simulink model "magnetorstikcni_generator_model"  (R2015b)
settings: Solver=VariableStepAuto  StartTime=0.0  StopTime=1  FixedStep=1e-3  RelTol=1e-3
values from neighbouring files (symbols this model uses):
  A = (pi*d_terf^2)/4    (= 5.02654824574e-05)    [parametry_magneto.m]    (also in P_016_80_parametry.m = 0.00020106192983)
  A_c = ((pi*D_c^2)/4)-((pi*d_c^2)/4)    [parametry_magneto.m]
  b = 2*b_p*m_t*ome    [parametry_magneto.m]    (also in P_016_80_parametry.m = 415.611533333)
  b_amp = 2*0.02*m_amp*ome_amp    (= 29.2857142857)    [parametry_magneto.m]    (also in piezoelektricky_genarator_parametry.m = 3.90920092413)
  d33 = 2e-9    (= 2e-09)    [parametry_magneto.m]    (also in P_016_80_parametry.m = 6.5e-10)
  delta_x = 4e-4    (= 0.0004)    [parametry_magneto.m]    (also in piezoelektricky_genarator_parametry.m)
  k = E*A/l_terf    (= 1005309649.15)    [parametry_magneto.m]    (also in P_016_80_parametry.m = 56000000)
  k_amp = F_in/delta_x    (= 6821500)    [parametry_magneto.m]    (also in piezoelektricky_genarator_parametry.m)
  L = (perm*(N_c^2)*A_c)/l_c    [parametry_magneto.m]
  l_terf = 0.025    [parametry_magneto.m]
  m = m_t+m_amp    (= 2.02300536849)    [parametry_magneto.m]    (also in piezoelektricky_genarator_parametry.m = m_eff+m_amp; P_016_80_parametry.m = 0.1804)
  N_c = N_c_row*floor(N_c/N_c_row)    [parametry_magneto.m]
  perm = 6.29e-6    (= 6.29e-06)    [parametry_magneto.m]
  Rc = 4*(ro_Cu*l_d)/(pi*d_d^2)    [parametry_magneto.m]
  Rz = 250    [parametry_magneto.m]

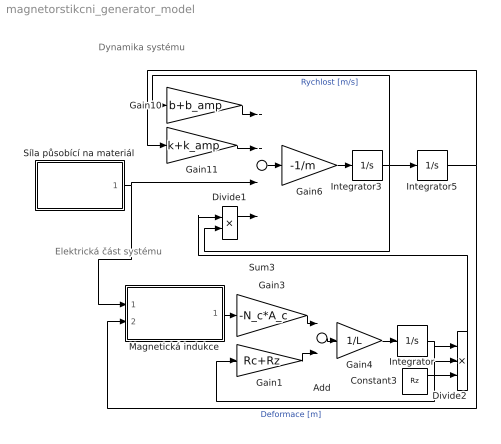
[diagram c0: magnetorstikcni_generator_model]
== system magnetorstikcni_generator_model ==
  note: Dynamika systému
  note: Elektrická část systému
  Add : Sum  Inputs=+-
  Constant3 : Constant  Value=Rz
  Divide1 : Product  Inputs=*/
  Divide2 : Product  Inputs=***
  Gain1 : Gain  Gain=Rc+Rz
  Gain10 : Gain  Gain=b+b_amp
  Gain11 : Gain  Gain=k+k_amp
  Gain3 : Gain  Gain=-N_c*A_c
  Gain4 : Gain  Gain=1/L
  Gain6 : Gain  Gain=-1/m
  Integrator : Integrator
  Integrator3 : Integrator  InitialCondition=1.5e-5
  Integrator5 : Integrator
  Magnetická indukce : Subsystem
  Sum3 : Sum  Inputs=++--
  Síla působící na materiál : Subsystem
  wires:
  Gain6/1 -> Integrator3/1
  Sum3/1 -> Gain6/1
  Gain10/1 -> Sum3/1
  Integrator3/1 -> Integrator5/1, Gain10/1, Divide1/2  "Rychlost [m/s]"
  Gain11/1 -> Sum3/2
  Integrator5/1 -> Gain11/1, Magnetická indukce/2(Deformace)  "Deformace [m]"
  Gain3/1 -> Add/1
  Add/1 -> Gain4/1
  Gain1/1 -> Add/2
  Gain4/1 -> Integrator/1
  Integrator/1 -> Divide2/2, Gain1/1, Divide2/1
  Constant3/1 -> Divide2/3
  Divide2/1 -> Divide1/1
  Magnetická indukce/1("derivace ") -> Gain3/1
  Divide1/1 -> Sum3/4
  Síla působící na materiál/1(Síla) -> Sum3/3, Magnetická indukce/1(Síla na Stack)

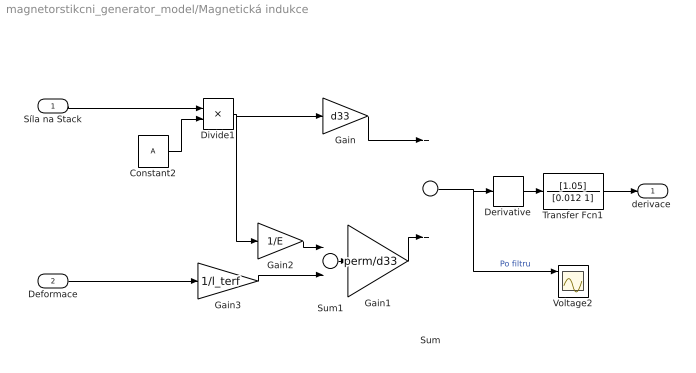
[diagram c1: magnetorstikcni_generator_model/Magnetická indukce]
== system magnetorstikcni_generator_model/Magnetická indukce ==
  Síla na Stack : Inport
  Deformace : Inport  Port=2
  Constant2 : Constant  Value=A
  Derivative : Derivative
  Divide1 : Product  Inputs=*/
  Gain : Gain  Gain=d33
  Gain1 : Gain  Gain=perm/d33
  Gain2 : Gain  Gain=1/E
  Gain3 : Gain  Gain=1/l_terf
  Sum : Sum
  Sum1 : Sum  Inputs=-+
  Transfer Fcn1 : TransferFcn  Numerator=[1.05]  Denominator=[0.012 1]
  Voltage2 : Scope  NumInputPorts=4
  "derivace " : Outport
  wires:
  Constant2/1 -> Divide1/2
  Gain/1 -> Sum/1
  Gain1/1 -> Sum/2
  Sum1/1 -> Gain1/1
  Gain3/1 -> Sum1/2
  Gain2/1 -> Sum1/1
  Derivative/1 -> Transfer Fcn1/1
  Sum/1 -> Voltage2/1, Derivative/1  "Po filtru"
  Divide1/1 -> Gain/1, Gain2/1
  Síla na Stack/1 -> Divide1/1
  Transfer Fcn1/1 -> "derivace "/1
  Deformace/1 -> Gain3/1

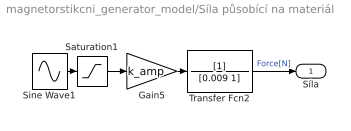
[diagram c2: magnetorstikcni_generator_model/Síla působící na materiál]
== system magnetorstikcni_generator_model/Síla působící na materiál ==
  Gain5 : Gain  Gain=k_amp
  Saturation1 : Saturate  UpperLimit=delta_x  LowerLimit=0
  Sine Wave1 : Sin  Amplitude=2*delta_x  Frequency=2*pi*2  SampleTime=0
  Transfer Fcn2 : TransferFcn  Denominator=[0.009 1]
  Síla : Outport
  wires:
  Gain5/1 -> Transfer Fcn2/1
  Sine Wave1/1 -> Saturation1/1
  Transfer Fcn2/1 -> Síla/1  "Force[N]"
  Saturation1/1 -> Gain5/1
